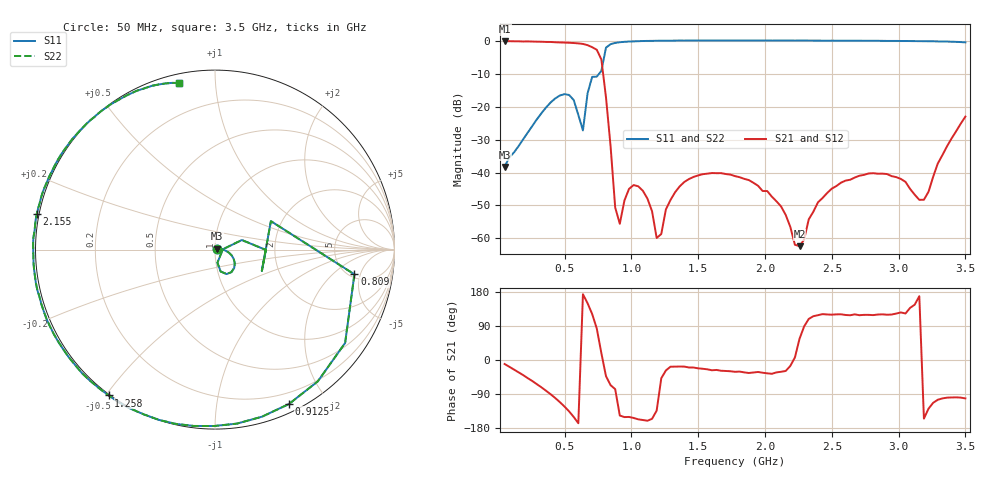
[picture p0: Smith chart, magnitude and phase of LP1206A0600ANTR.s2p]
!Instrument: 	"HEWLETT PACKARD,8720ES,US39172150,7.62 "
!	AVX THIN FILM OPERATION
!	LP1206 High Performance Low Pass Filters
!	P/N LP1206A0600ANTR  12 May 2019
# MHz S dB R 50
!  Frq	S11(dB)	S11(deg)	S21(dB)	S21(deg)	S12(dB)	S12(deg)	S22(dB)	S22(deg)
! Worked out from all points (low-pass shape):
!   101 points, 50 MHz to 3.5 GHz, reference 50 ohm
!   highest |S21| = -0.08 dB at 50 MHz (marker M1); lowest = -62.4 dB at 2.258 GHz (marker M2)
!   |S21| within 3 dB of the highest: start of sweep to 744.6 MHz
!   lowest |S11| = -38.3 dB at 50 MHz (marker M3), VSWR 1.02, Z = 51.1 + j0.512 ohm
!   |S11| at or under -10 dB: start of sweep to 757 MHz
!   |S22| runs from -38.3 to 0.1 dB; largest |S21 - S12| = 0
!   S11 on the Smith chart (normalised r, x): 50 MHz: 1.02, +0.01; 809 MHz: 5.48, -4.00; 912.5 MHz: 0.08, -1.58; 1.258 GHz: -0.00, -0.51; 2.155 GHz: -0.01, +0.10; 3.5 GHz: 0.04, +0.81
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50  -38.29 24.3  -0.08 -10.6  -0.08 -10.6  -38.29 24.3
395  -18.70 -26.2  -0.33 -90.5  -0.33 -90.5  -18.70 -26.2
533  -16.43 -64.7  -0.57 -135.7  -0.57 -135.7  -16.43 -64.7
636.5  -27.21 2.2  -0.92 173.5  -0.92 173.5  -27.21 2.2
671  -15.98 19.6  -1.30 149.9  -1.30 149.9  -15.98 19.6
740  -10.85 -24.5  -2.69 83.2  -2.69 83.2  -10.85 -24.5
774.5  -9.13 27.0  -5.64 17.9  -5.64 17.9  -9.13 27.0
809  -2.06 -10.1  -17.13 -42.6  -17.13 -42.6  -2.06 -10.1
878  -0.62 -52.0  -50.64 -76.9  -50.64 -76.9  -0.62 -52.0
912.5  -0.41 -64.4  -55.58 -146.5  -55.58 -146.5  -0.41 -64.4
1016  -0.15 -90.3  -43.81 -152.9  -43.81 -152.9  -0.15 -90.3
1223  0.05 -122.1  -58.68 -48.3  -58.68 -48.3  0.05 -122.1
1257.5  0.05 -126.1  -51.21 -27.6  -51.21 -27.6  0.05 -126.1
1430  0.10 -143.6  -41.99 -19.8  -41.99 -19.8  0.10 -143.6
1775  0.13 -169.5  -41.09 -31.2  -41.09 -31.2  0.13 -169.5
2154.5  0.11 168.6  -52.87 -28.9  -52.87 -28.9  0.11 168.6
2258  0.10 163.2  -62.38 55.8  -62.38 55.8  0.10 163.2
2361.5  0.08 158.0  -51.92 115.6  -51.92 115.6  0.08 158.0
2603  0.06 146.5  -42.45 118.8  -42.45 118.8  0.06 146.5
2948  -0.01 130.8  -41.10 119.9  -41.10 119.9  -0.01 130.8
3189.5  -0.09 119.5  -48.27 -154.7  -48.27 -154.7  -0.09 119.5
3500  -0.45 102.1  -23.01 -101.4  -23.01 -101.4  -0.45 102.1
